
DATA_BLOCK DB3492
TITLE=
VERSION : 0.1

STRUCT
   CM_ID : STRING  [8 ] := '=PRM'; //COMPOSITE MACHINE
   STATION_ID : STRING  [8 ] := '++OP10'; //STATION - TRATTO - ZONE
   ELEMENT_ID : STRING  [8 ] := '+81CLM82'; //ELEMENT
   DB_ID : INT := 0 ; //DB SIZE OR TYPE
   PART_STYLE : STRING  [12 ]; //PART STYLE ON LAST STATION
   ACT_CYCLE_TIME : INT ; //ACTUAL CYCLE TIME FOR THIS STYLE
   COUNT_GOOD : INT ; //COUNTER GOOD PIECES
   COUNT_SCRAP : INT ; //COUNTER SCRAP PIECES
   SPARE_00 : ARRAY  [0 .. 15 ] OF //SPARE INTEGER
   INT ;
   SPARE_01 : ARRAY  [0 .. 17 ] OF //SPARE INTEGER
   INT ;
   CODE_EVENT : ARRAY  [0 .. 7 ] OF //CODE EVENT - EXTENDED FAULT CODE DIAGNOSTIC
   INT ;
   EVENT : STRUCT
E0000 : BOOL ; //+81CLM82-B49N; MS. ERRORE GENERALE TEMPERATURA;1
E0001 : BOOL ; //+81CLM82-B49N; MS. AVVERTENZE GENERALE TEMPERATURA;2
E0002 : BOOL ; //+81CLM82-B49N; MS. TEMPERATURA OK;58
E0003 : BOOL ; //+81CLM82-B49N; MS. SM_03 TEMPERATURA;58
E0004 : BOOL ; //+81CLM82-B49N; MS. SM_04 TEMPERATURA;58
E0005 : BOOL ; //+81CLM82-B49N; MS. SM_05 TEMPERATURA;58
E0006 : BOOL ; //+81CLM82-B49N; MS. SM_06 TEMPERATURA;58
E0007 : BOOL ; //+81CLM82-B49N; MS. SM_07 TEMPERATURA;58
E0008 : BOOL ; //+81CLM82-B49N; MS. L03 AVVERTENZE MAXIMO TEMPERATURA;2
E0009 : BOOL ; //+81CLM82-B49N; MS. L02 AVVERTENZE MINIMO TEMPERATURA;2
E0010 : BOOL ; //+81CLM82-B49N; MS. SM_12 TEMPERATURA;58
E0011 : BOOL ; //+81CLM82-B49N; MS. SM_13 TEMPERATURA;58
E0012 : BOOL ; //+81CLM82-B49N; MS. SM_14 TEMPERATURA;58
E0013 : BOOL ; //+81CLM82-B49N; MS. SM_15 TEMPERATURA;58
E0014 : BOOL ; //+81CLM82-B49N; MS. SM_16 TEMPERATURA;58
E0015 : BOOL ; //+81CLM82-B49N; MS. TEMPERATURA TROPPO ALTA;58
E0016 : BOOL ; //+81CLM82-B49N; ME. L04 ERRORE MAXIMO TEMPERATURA;1
E0017 : BOOL ; //+81CLM82-B49N; ME. L01 AVVERTENZE MINIMO TEMPERATURA;1
E0018 : BOOL ; //+81CLM82-B49N; ME. FM_02 TEMPERATURA;58
E0019 : BOOL ; //+81CLM82-B49N; ME. FM_03 TEMPERATURA;58
E0020 : BOOL ; //+81CLM82-B49N; ME. FM_04 TEMPERATURA;58
E0021 : BOOL ; //+81CLM82-B49N; ME. FM_05 TEMPERATURA;58
E0022 : BOOL ; //+81CLM82-B49N; ME. FM_06 TEMPERATURA;58
E0023 : BOOL ; //+81CLM82-B49N; ME. FM_07 TEMPERATURA;58
E0024 : BOOL ; //+81CLM82-B49N; ME. FM_10 TEMPERATURA;58
E0025 : BOOL ; //+81CLM82-B49N; ME. FM_11 TEMPERATURA;58
E0026 : BOOL ; //+81CLM82-B49N; ME. FM_12 TEMPERATURA;58
E0027 : BOOL ; //+81CLM82-B49N; ME. FM_13 TEMPERATURA;58
E0028 : BOOL ; //+81CLM82-B49N; ME. FM_14 TEMPERATURA;58
E0029 : BOOL ; //+81CLM82-B49N; ME. FM_15 TEMPERATURA;58
E0030 : BOOL ; //+81CLM82-B49N; ME. FM_16 TEMPERATURA;58
E0031 : BOOL ; //+81CLM82-B49N; ME. FM_17 TEMPERATURA;58
E0032 : BOOL ; //+81CLM82-B49N; MS. ERRORE GENERALE UMIDITA;1
E0033 : BOOL ; //+81CLM82-B49N; MS. AVVERTENZE GENERALE UMIDITA;2
E0034 : BOOL ; //+81CLM82-B49N; MS. TEMPERATURA OK UMIDITA;58
E0035 : BOOL ; //+81CLM82-B49N; MS. SM_03 UMIDITA;58
E0036 : BOOL ; //+81CLM82-B49N; MS. SM_04 UMIDITA;58
E0037 : BOOL ; //+81CLM82-B49N; MS. SM_05 UMIDITA;58
E0038 : BOOL ; //+81CLM82-B49N; MS. SM_06 UMIDITA;58
E0039 : BOOL ; //+81CLM82-B49N; MS. SM_07 UMIDITA;58
E0040 : BOOL ; //+81CLM82-B49N; MS. L03 AVVERTENZE MAXIMO UMIDITA;2
E0041 : BOOL ; //+81CLM82-B49N; MS. L02 AVVERTENZE MINIMO UMIDITA;2
E0042 : BOOL ; //+81CLM82-B49N; MS. SM_12 UMIDITA;58
E0043 : BOOL ; //+81CLM82-B49N; MS. SM_13 UMIDITA;58
E0044 : BOOL ; //+81CLM82-B49N; MS. SM_14 UMIDITA;58
E0045 : BOOL ; //+81CLM82-B49N; MS. SM_15 UMIDITA;58
E0046 : BOOL ; //+81CLM82-B49N; MS. SM_16 UMIDITA;58
E0047 : BOOL ; //+81CLM82-B49N; MS. TEMPERATURA TROPPO ALTA;58
E0048 : BOOL ; //+81CLM82-B49N; ME. L04 ERRORE MAXIMO UMIDITA;1
E0049 : BOOL ; //+81CLM82-B49N; ME. L01 ERRORE MINIMO UMIDITA;1
E0050 : BOOL ; //+81CLM82-B49N; ME. FM_02 UMIDITA;58
E0051 : BOOL ; //+81CLM82-B49N; ME. FM_03 UMIDITA;58
E0052 : BOOL ; //+81CLM82-B49N; ME. FM_04 UMIDITA;58
E0053 : BOOL ; //+81CLM82-B49N; ME. FM_05 UMIDITA;58
E0054 : BOOL ; //+81CLM82-B49N; ME. FM_06 UMIDITA;58
E0055 : BOOL ; //+81CLM82-B49N; ME. FM_07 UMIDITA;58
E0056 : BOOL ; //+81CLM82-B49N; ME. FM_10 UMIDITA;58
E0057 : BOOL ; //+81CLM82-B49N; ME. FM_11 UMIDITA;58
E0058 : BOOL ; //+81CLM82-B49N; ME. FM_12 UMIDITA;58
E0059 : BOOL ; //+81CLM82-B49N; ME. FM_13 UMIDITA;58
E0060 : BOOL ; //+81CLM82-B49N; ME. FM_14 UMIDITA;58
E0061 : BOOL ; //+81CLM82-B49N; ME. FM_15 UMIDITA;58
E0062 : BOOL ; //+81CLM82-B49N; ME. FM_16 UMIDITA;58
E0063 : BOOL ; //+81CLM82-B49N; ME. FM_17 UMIDITA;58
END_STRUCT;
END_STRUCT;
BEGIN
CM_ID := '=PRM';
STATION_ID := '++OP10';
ELEMENT_ID := '+81CLM82';
DB_ID := 0 ;
PART_STYLE := '';
ACT_CYCLE_TIME := 0;
COUNT_GOOD := 0;
COUNT_SCRAP := 0;
SPARE_00[0] := 0;
SPARE_00[1] := 0;
SPARE_00[2] := 0;
SPARE_00[3] := 0;
SPARE_00[4] := 0;
SPARE_00[5] := 0;
SPARE_00[6] := 0;
SPARE_00[7] := 0;
SPARE_00[8] := 0;
SPARE_00[9] := 0;
SPARE_00[10] := 0;
SPARE_00[11] := 0;
SPARE_00[12] := 0;
SPARE_00[13] := 0;
SPARE_00[14] := 0;
SPARE_00[15] := 0;
SPARE_01[0] := 0;
SPARE_01[1] := 0;
SPARE_01[2] := 0;
SPARE_01[3] := 0;
SPARE_01[4] := 0;
SPARE_01[5] := 0;
SPARE_01[6] := 0;
SPARE_01[7] := 0;
SPARE_01[8] := 0;
SPARE_01[9] := 0;
SPARE_01[10] := 0;
SPARE_01[11] := 0;
SPARE_01[12] := 0;
SPARE_01[13] := 0;
SPARE_01[14] := 0;
SPARE_01[15] := 0;
SPARE_01[16] := 0;
SPARE_01[17] := 0;
CODE_EVENT[0] := 0;
CODE_EVENT[1] := 0;
CODE_EVENT[2] := 0;
CODE_EVENT[3] := 0;
CODE_EVENT[4] := 0;
CODE_EVENT[5] := 0;
CODE_EVENT[6] := 0;
CODE_EVENT[7] := 0;
EVENT.E0000 := FALSE;
EVENT.E0001 := FALSE;
EVENT.E0002 := FALSE;
EVENT.E0003 := FALSE;
EVENT.E0004 := FALSE;
EVENT.E0005 := FALSE;
EVENT.E0006 := FALSE;
EVENT.E0007 := FALSE;
EVENT.E0008 := FALSE;
EVENT.E0009 := FALSE;
EVENT.E0010 := FALSE;
EVENT.E0011 := FALSE;
EVENT.E0012 := FALSE;
EVENT.E0013 := FALSE;
EVENT.E0014 := FALSE;
EVENT.E0015 := FALSE;
EVENT.E0016 := FALSE;
EVENT.E0017 := FALSE;
EVENT.E0018 := FALSE;
EVENT.E0019 := FALSE;
EVENT.E0020 := FALSE;
EVENT.E0021 := FALSE;
EVENT.E0022 := FALSE;
EVENT.E0023 := FALSE;
EVENT.E0024 := FALSE;
EVENT.E0025 := FALSE;
EVENT.E0026 := FALSE;
EVENT.E0027 := FALSE;
EVENT.E0028 := FALSE;
EVENT.E0029 := FALSE;
EVENT.E0030 := FALSE;
EVENT.E0031 := FALSE;
EVENT.E0032 := FALSE;
EVENT.E0033 := FALSE;
EVENT.E0034 := FALSE;
EVENT.E0035 := FALSE;
EVENT.E0036 := FALSE;
EVENT.E0037 := FALSE;
EVENT.E0038 := FALSE;
EVENT.E0039 := FALSE;
EVENT.E0040 := FALSE;
EVENT.E0041 := FALSE;
EVENT.E0042 := FALSE;
EVENT.E0043 := FALSE;
EVENT.E0044 := FALSE;
EVENT.E0045 := FALSE;
EVENT.E0046 := FALSE;
EVENT.E0047 := FALSE;
EVENT.E0048 := FALSE;
EVENT.E0049 := FALSE;
EVENT.E0050 := FALSE;
EVENT.E0051 := FALSE;
EVENT.E0052 := FALSE;
EVENT.E0053 := FALSE;
EVENT.E0054 := FALSE;
EVENT.E0055 := FALSE;
EVENT.E0056 := FALSE;
EVENT.E0057 := FALSE;
EVENT.E0058 := FALSE;
EVENT.E0059 := FALSE;
EVENT.E0060 := FALSE;
EVENT.E0061 := FALSE;
EVENT.E0062 := FALSE;
EVENT.E0063 := FALSE;
END_DATA_BLOCK
